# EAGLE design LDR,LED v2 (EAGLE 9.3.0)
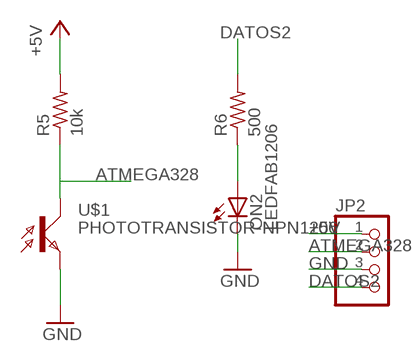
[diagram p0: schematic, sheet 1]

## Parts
JP2  PINHD-1X4/90  [1X04/90]
ON2  LEDFAB1206  [LED1206FAB]
R5  10k  RES-US1206FAB  [R1206FAB]
R6  500  RES-US1206FAB  [R1206FAB]
U$1  PHOTOTRANSISTOR-NPN1206  [OP1206]

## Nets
+5V: JP2.1 R5.2
ATMEGA328: JP2.2 R5.1 U$1.COLLECTOR(C)
DATOS2: JP2.4 R6.2
GND: JP2.3 ON2.2(C) U$1.EMITTER(E)
N$6: ON2.1(A) R6.1

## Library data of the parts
JP2 = pinhead:PINHD-1X4: PIN HEADER
ON2 = fab:LED: LED
R5 R6 = fab:RES-US: Resistor (US Symbol)
U$1 = fab:PHOTOTRANSISTOR-NPN

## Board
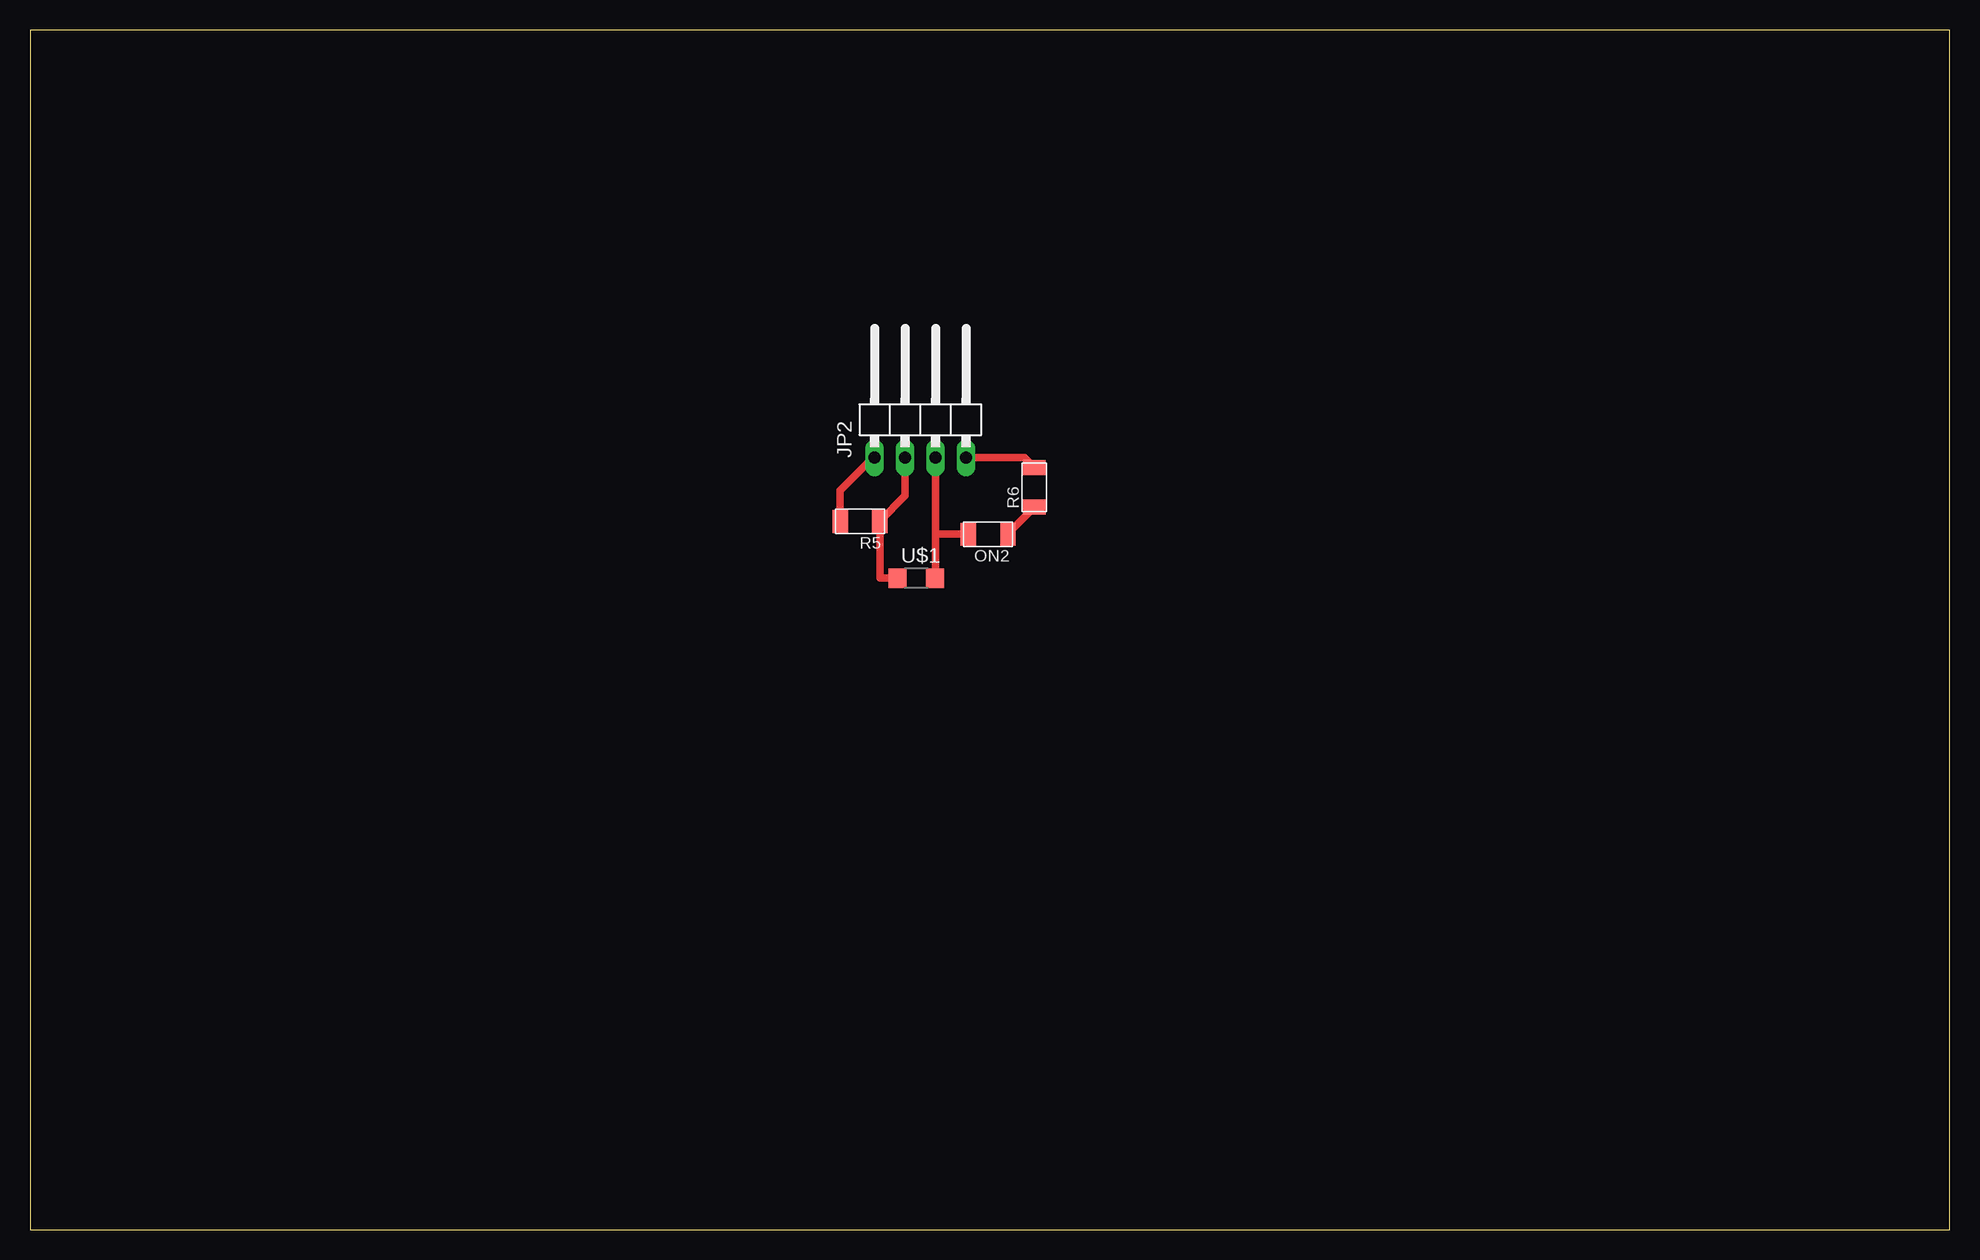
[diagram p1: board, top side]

Size 160 x 100 mm. Coordinates in mm from the lower left corner, seen from the top.
Outline: 0,0 160,0 160,100 0,100 0,0
Copper layers (1*16): Top 0.035mm / dielectric 1.5mm / Bottom 0.035mm
Design rules "default": minimum track width 6mil, minimum drill 0.35mm, track to track 6mil, track to pad 6mil, pad to pad 6mil, via to via 6mil, smd to smd 6mil, copper to edge 40mil, drill to drill 6mil, minimum pad ring 10mil, minimum via ring 8mil, stop-mask expansion 4mil, vias tented up to drill 0mil, thermal gap 10mil

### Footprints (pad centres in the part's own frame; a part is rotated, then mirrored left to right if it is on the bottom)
1X04/90 = drill 1.016 long: 1 -3.81,-3.81; 2 -1.27,-3.81; 3 1.27,-3.81; 4 3.81,-3.81
LED1206FAB = smd 1.27 x 1.905: 1 -1.651,0; 2 1.651,0
R1206FAB = smd 1.27 x 1.905: 1 -1.651,0; 2 1.651,0
OP1206 = smd 1.5 x 1.6: COLLECTOR -1.55,0; EMITTER 1.55,0

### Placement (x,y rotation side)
JP2  74.22,68.15 0 top
ON2  79.86,57.96 180 top
R5  69.19,59.03 180 top
R6  83.71,61.88 90 top
U$1  73.87,54.3 0 top

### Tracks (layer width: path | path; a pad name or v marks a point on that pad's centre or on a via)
+5V
  Top 0.61: R5.2 67.54,61.59 70.29,64.34 JP2.1
ATMEGA328
  Top 0.61: JP2.2 72.95,61.17 70.84,59.06 R5.1 70.84,54.3 U$1.COLLECTOR
DATOS2
  Top 0.61: JP2.4 82.9,64.34 R6.2
GND
  Top 0.61: JP2.3 75.49,57.96 | ON2.2 75.49,57.96 | 75.49,57.96 75.49,54.36 U$1.EMITTER
N$6
  Top 0.61: R6.1 81.51,58.02 ON2.1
